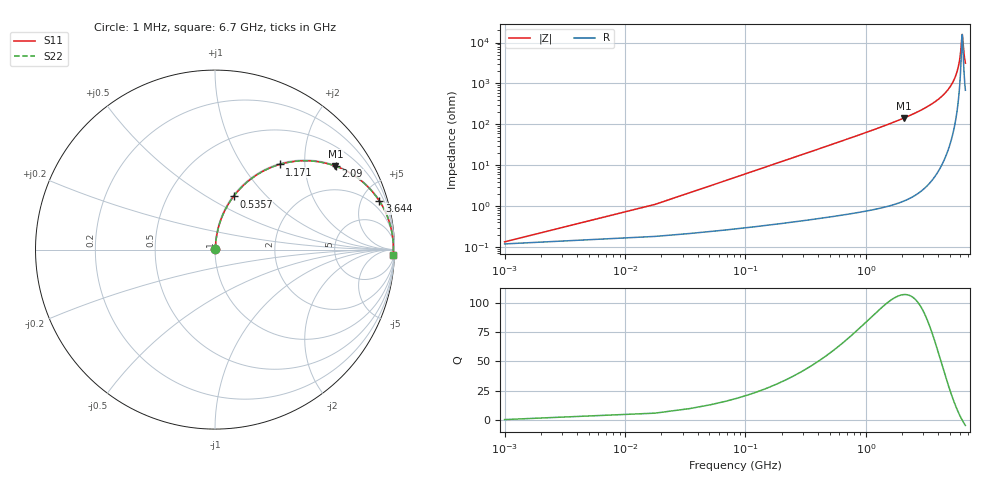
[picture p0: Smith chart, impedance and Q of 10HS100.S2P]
! Coilcraft 1008HS-100 Chip Inductor
! 02 July 2002
# MHZ S MA R 50
!Freq  MagS11  AngS11  MagS21  AngS21  MagS12  AngS12  MagS22  AngS22
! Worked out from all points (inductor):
!   402 points, 1 MHz to 6.7 GHz, reference 50 ohm
!   read as one part in series: L = 9.8 nH near 34.42 MHz
!   highest Q = 107 at 2.073 GHz (marker M1), where L = 11 nH
!   self-resonance near 6.301 GHz
!   S11 on the Smith chart (normalised r, x): 1 MHz: 1.00, +0.00; 535.7 MHz: 1.01, +0.66; 1.171 GHz: 1.02, +1.49; 2.09 GHz: 1.03, +2.89; 3.644 GHz: 1.10, +6.74; 6.7 GHz: 15, -61
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1  0.001344 27.2  0.9988 -0.0  0.9988 -0.0  0.001344 27.2
51.13  0.03149 83.8  0.9971 -1.8  0.9971 -1.8  0.03149 83.8
84.55  0.05193 83.9  0.9959 -3.0  0.9959 -3.0  0.05193 83.9
117.97  0.07232 83.4  0.9943 -4.1  0.9943 -4.1  0.07232 83.4
184.81  0.1128 81.7  0.99 -6.5  0.99 -6.5  0.1128 81.7
268.36  0.1627 79.2  0.9825 -9.4  0.9825 -9.4  0.1627 79.2
535.72  0.3138 70.7  0.9442 -18.3  0.9442 -18.3  0.3138 70.7
1120.57  0.5772 54.1  0.8101 -35.3  0.8101 -35.3  0.5772 54.1
1170.7  0.5951 52.8  0.7971 -36.5  0.7971 -36.5  0.5951 52.8
2073.04  0.8161 34.8  0.5703 -54.7  0.5703 -54.7  0.8161 34.8
2089.75  0.8188 34.5  0.5664 -55.0  0.5664 -55.0  0.8188 34.5
2240.14  0.8412 32.2  0.5329 -57.3  0.5329 -57.3  0.8412 32.2
3359.71  0.9414 19.0  0.3259 -70.3  0.3259 -70.3  0.9414 19.0
3643.78  0.9549 16.5  0.2835 -72.7  0.2835 -72.7  0.9549 16.5
4479.28  0.98 10.1  0.1761 -78.4  0.1761 -78.4  0.98 10.1
5130.97  0.9895 6.1  0.106 -81.3  0.106 -81.3  0.9895 6.1
5598.85  0.9928 3.5  0.06127 -81.5  0.06127 -81.5  0.9928 3.5
5999.89  0.9938 1.5  0.02623 -75.6  0.02623 -75.6  0.9938 1.5
6300.67  0.9937 0.0  0.006311 -4.8  0.006311 -4.8  0.9937 0.0
6350.8  0.9936 -0.2  0.007269 28.8  0.007269 28.8  0.9936 -0.2
6534.61  0.9932 -1.0  0.01928 68.9  0.01928 68.9  0.9932 -1.0
6700  0.9926 -1.8  0.03164 75.7  0.03164 75.7  0.9926 -1.8
